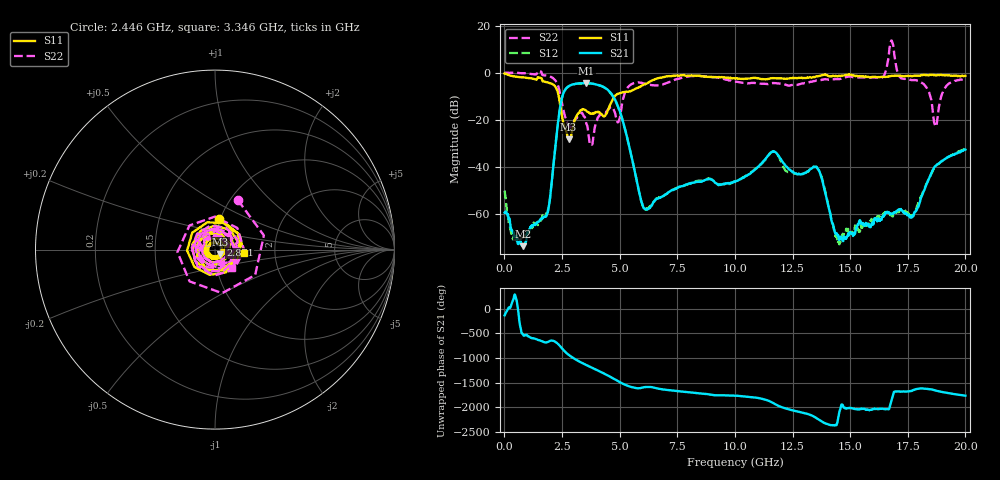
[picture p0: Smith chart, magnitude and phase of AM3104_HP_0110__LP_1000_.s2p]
!Created with skrf (http://scikit-rf.org).
# Hz S RI R 50.0
!freq ReS11 ImS11 ReS21 ImS21 ReS12 ImS12 ReS22 ImS22
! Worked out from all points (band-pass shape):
!   1601 points, 10 MHz to 20 GHz, reference 50 ohm
!   highest |S21| = -4.45 dB at 3.558 GHz (marker M1); lowest = -73.7 dB at 797.1 MHz (marker M2)
!   |S21| within 3 dB of the highest: 2.626 GHz to 4.501 GHz (1.875 GHz wide, 52.6 % of centre)
!   lowest |S11| = -28.2 dB at 2.784 GHz (marker M3), VSWR 1.08, Z = 52.9 - j2.71 ohm
!   |S11| at or under -10 dB: 2.357 GHz to 4.789 GHz (2.432 GHz wide, 68.1 % of centre)
!   |S22| runs from -30.6 to 13.7 dB; largest |S21 - S12| = 0.044
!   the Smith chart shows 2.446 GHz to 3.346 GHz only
!   S11 on the Smith chart (normalised r, x): 2.446 GHz: 0.98, +0.34; 2.871 GHz: 1.06, +0.06; 3.346 GHz: 1.38, -0.05
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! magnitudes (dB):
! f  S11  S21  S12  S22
! 10 MHz  -0.4  -59.5  -50.1  -0.1
! 384.8 MHz  -1.5  -67.5  -70.9  -0.1
! 797.1 MHz  -2.0  -73.7  -70.2  -0.2
! 1.884 GHz  -4.2  -59.3  -58.7  -1.4
! 2.446 GHz  -15.4  -13.1  -13.2  -10.4
! 2.784 GHz  -28.2  -5.8  -5.9  -22.6
! 2.871 GHz  -27.9  -5.4  -5.4  -23.2
! 3.346 GHz  -15.8  -4.5  -4.6  -17.0
! 3.558 GHz  -16.3  -4.5  -4.5  -21.8
! 3.771 GHz  -17.4  -4.6  -4.7  -30.3
! 4.858 GHz  -9.4  -12.7  -12.7  -19.7
! 6.044 GHz  -5.1  -57.5  -57.0  -4.6
! 6.682 GHz  -2.3  -53.4  -53.1  -5.4
! 10.01 GHz  -2.5  -46.5  -46.2  -3.9
! 11.64 GHz  -2.4  -33.5  -33.5  -4.4
! 13.34 GHz  -2.1  -40.6  -40.6  -3.9
! 14.53 GHz  -1.4  -71.1  -72.9  -2.8
! 16.68 GHz  -1.6  -59.4  -59.7  7.3
! 17.69 GHz  -1.5  -61.0  -61.4  -3.2
! 18.7 GHz  -1.2  -39.7  -39.7  -22.6
! 19.14 GHz  -1.1  -36.6  -36.6  -6.2
! 20 GHz  -1.4  -32.7  -32.1  -2.6
